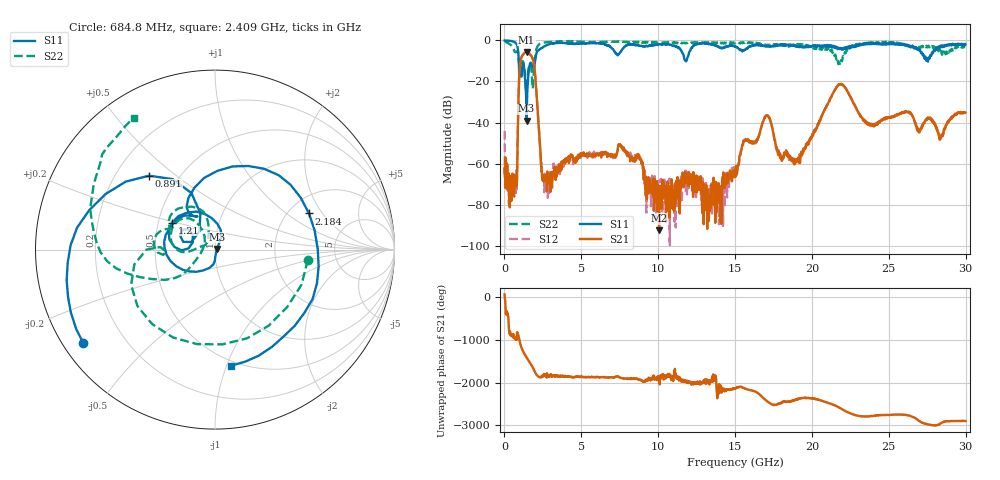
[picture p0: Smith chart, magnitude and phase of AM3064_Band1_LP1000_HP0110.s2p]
# Hz S DB R 50.0
!freq dBS11 angS11 dBS21 angS21 dBS12 angS12 dBS22 angS22
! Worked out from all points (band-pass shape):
!   1600 points, 10 MHz to 29.98 GHz, reference 50 ohm
!   highest |S21| = -5.61 dB at 1.435 GHz (marker M1); lowest = -92.5 dB at 10.06 GHz (marker M2)
!   |S21| within 3 dB of the highest: 1.091 GHz to 1.825 GHz (734.1 MHz wide, 50.4 % of centre)
!   lowest |S11| = -39.1 dB at 1.435 GHz (marker M3), VSWR 1.02, Z = 51 + j0.419 ohm
!   |S11| at or under -10 dB: 931.6 MHz to 1.994 GHz (1.062 GHz wide, 72.6 % of centre); 11.79355 GHz to 11.83792 GHz (44.37 MHz wide, 0.376 % of centre); 27.52379 GHz to 27.55134 GHz (27.56 MHz wide, 0.1 % of centre)
!   |S22| runs from -24.6 to -0.3 dB; largest |S21 - S12| = 0.0065
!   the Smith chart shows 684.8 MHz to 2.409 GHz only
!   S11 on the Smith chart (normalised r, x): 684.8 MHz: 0.06, -0.32; 891 MHz: 0.34, +0.40; 1.21 GHz: 0.59, +0.19; 2.184 GHz: 2.56, +1.51; 2.409 GHz: 0.46, -1.04
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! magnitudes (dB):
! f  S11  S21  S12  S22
! 10 MHz  -0.1  -62.4  -44.1  -0.3
! 684.8 MHz  -0.9  -71.5  -68.5  -5.7
! 891 MHz  -5.2  -35.6  -35.5  -6.8
! 1.21 GHz  -11.0  -7.0  -6.9  -10.3
! 1.435 GHz  -39.1  -5.6  -5.6  -23.6
! 1.884 GHz  -13.6  -10.1  -10.1  -18.3
! 2.184 GHz  -5.0  -36.9  -37.0  -2.5
! 2.409 GHz  -3.7  -63.8  -61.9  -1.3
! 2.859 GHz  -2.1  -64.7  -73.8  -0.8
! 5.015 GHz  -1.4  -55.8  -56.0  -0.6
! 7.564 GHz  -5.5  -51.5  -51.1  -0.6
! 10 GHz  -2.0  -70.9  -71.9  -0.9
! 10.06 GHz  -2.0  -92.5  -73.8  -1.0
! 13.88 GHz  -3.1  -70.7  -73.9  -1.2
! 15 GHz  -3.1  -65.2  -66.0  -1.4
! 17.03 GHz  -3.0  -36.5  -36.4  -2.5
! 18.02 GHz  -1.8  -57.5  -56.5  -2.2
! 19.99 GHz  -3.1  -46.8  -46.6  -3.1
! 21.83 GHz  -3.9  -21.3  -21.3  -12.0
! 25 GHz  -1.3  -37.6  -37.4  -1.1
! 28.39 GHz  -2.7  -47.1  -47.9  -5.1
! 29.98 GHz  -1.8  -35.2  -35.5  -3.2
